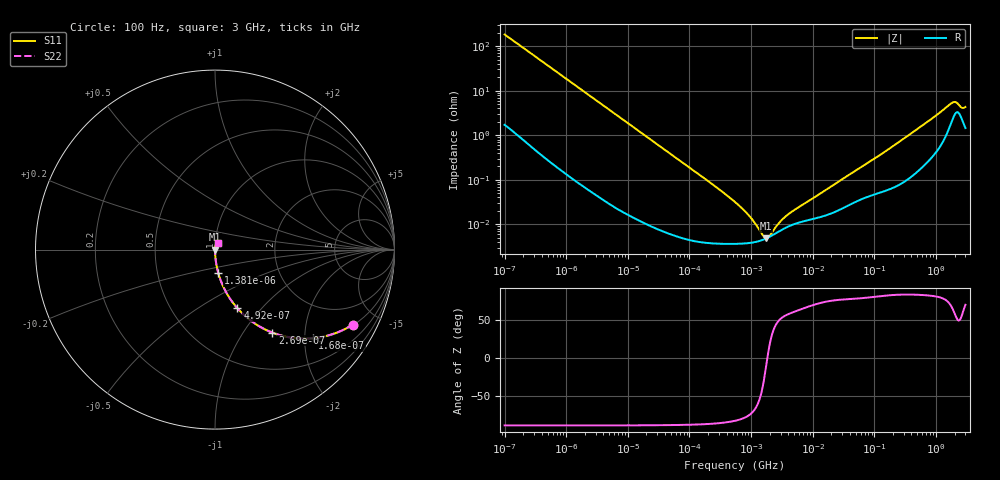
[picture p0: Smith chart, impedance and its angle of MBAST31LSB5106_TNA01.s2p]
! MBAST31LSB5106_TNA01  S-PARAMETER MODEL  ( Standard Model )
! Model Generated by TAIYO YUDEN Corporation (http://www.ty-top.com)
! Version 1.0
! TAIYO YUDEN Control No. 220601
! Copyright(c) 2012 TAIYO YUDEN CO.,LTD. All Rights Reserved.
! Product Description (link to TY-COMPAS)
! https://ds.yuden.co.jp/TYCOMPAS/or/detail?pn=MBAST31LSB5106KTNA01&u=M
! Products Name : Multilayer Ceramic Capacitors
! Characteristics :
!  Capacitance : 10 [uF] , Rated Voltage : 25 [V] , TCC : X5R
!  Case Size : 3.2 x 1.6 / 0.126 x 0.063 [mm/inch] , Thickness : 1.6 / 0.063 [mm/inch]
!  (Conditions: Temperature = 25 [degC] , DC Bias Voltage = 0 [V])
! External Node Assignments :
!  1  o---| |---o  2
! GND o---------o GND
! Frequency Range : 100Hz  -  3GHz  [ 401 STEP ]
# MHZ S RI R 50
! Freq[MHz].  S11 Real  S11 Imag  S21 Real  S21 Imag  S12 Real  S12 Imag  S22 Real  S22 Imag
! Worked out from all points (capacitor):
!   401 points, 100 Hz to 3 GHz, reference 50 ohm
!   read as one part in series: C = 8.69 uF near 109 Hz
!   lowest |Z| = 4.89 mohm at 1.751 MHz (marker M1)
!   series resonance near 1.836 MHz, so ESL is about 870 pH
!   S11 on the Smith chart (normalised r, x): 100 Hz: 1.03, -3.66; 168 Hz: 1.02, -2.19; 269 Hz: 1.01, -1.37; 492 Hz: 1.01, -0.75; 1.381 kHz: 1.00, -0.27; 3 GHz: 1.03, +0.08
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0.0001  0.7677 -0.4177  0.2323 0.4177  0.2323 0.4177  0.7677 -0.4177
0.000168  0.5448 -0.4936  0.4552 0.4936  0.4552 0.4936  0.5448 -0.4936
0.000269  0.3199 -0.4624  0.6801 0.4624  0.6801 0.4624  0.3199 -0.4624
0.000492  0.1253 -0.3273  0.8747 0.3273  0.8747 0.3273  0.1253 -0.3273
0.000789  0.0534 -0.2213  0.9466 0.2213  0.9466 0.2213  0.0534 -0.2213
0.001381  0.0186 -0.1315  0.9814 0.1315  0.9814 0.1315  0.0186 -0.1315
0.001788  0.0114 -0.1025  0.9886 0.1025  0.9886 0.1025  0.0114 -0.1025
0.005476  0.00142 -0.034  0.9986 0.034  0.9986 0.034  0.00142 -0.034
0.031977  0.00011 -0.00587  0.9999 0.00587  0.9999 0.00587  0.00011 -0.00587
0.221826  3.82e-05 -0.000841  1 0.000841  1 0.000841  3.82e-05 -0.000841
0.547723  3.64e-05 -0.000315  1 0.000315  1 0.000315  3.64e-05 -0.000315
0.806856  3.73e-05 -0.000189  1 0.000189  1 0.000189  3.73e-05 -0.000189
1.188587  4.02e-05 -9.16e-05  1 9.16e-05  1 9.16e-05  4.02e-05 -9.16e-05
1.75092  4.8e-05 -9.38e-06  1 9.38e-06  1 9.38e-06  4.8e-05 -9.38e-06
2.69274  6.64e-05 7.23e-05  0.9999 -7.23e-05  0.9999 -7.23e-05  6.64e-05 7.23e-05
4.323298  9.32e-05 0.000156  0.9999 -0.000156  0.9999 -0.000156  9.32e-05 0.000156
9.794414  0.00013 0.000351  0.9999 -0.000351  0.9999 -0.000351  0.00013 0.000351
175.1444  0.000632 0.00495  0.9994 -0.00495  0.9994 -0.00495  0.000632 0.00495
1789.813  0.0217 0.0467  0.9783 -0.0467  0.9783 -0.0467  0.0217 0.0467
2036.508  0.0311 0.0444  0.9689 -0.0444  0.9689 -0.0444  0.0311 0.0444
2636.591  0.0233 0.0329  0.9767 -0.0329  0.9767 -0.0329  0.0233 0.0329
3000  0.0159 0.0394  0.9841 -0.0394  0.9841 -0.0394  0.0159 0.0394
